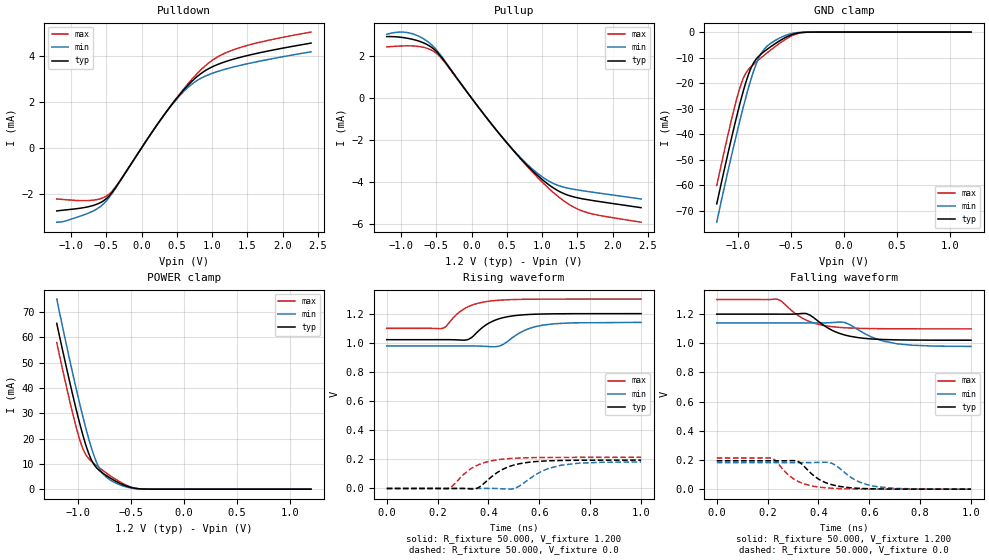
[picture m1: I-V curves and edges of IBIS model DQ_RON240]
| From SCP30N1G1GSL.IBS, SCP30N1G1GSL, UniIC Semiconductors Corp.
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|   Model DQ_RON240
[Model] DQ_RON240
Model_type I/O
Vinl =  0.500V
Vinh =  0.700V
Vmeas =  0.600V
Rref =  50.000
Vref =  0.600V
C_comp   1.373pF   1.353pF   1.403pF
[Model Spec]
Vinh   0.700V   0.670V   0.750V
Vinl   0.500V   0.470V   0.550V
Vmeas   0.600V   0.570V   0.650V
Vref   0.600V   0.570V   0.650V
Rref   50.000   NA   NA
[Temperature Range]   25.000   85.000   -40.000
[Voltage Range]   1.200V   1.140V   1.300V
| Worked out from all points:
|   slope of the pulldown table from 0 to 0.18 V, typ, clamps not added: 216 ohm
|   slope of the pullup table from 0 to 0.18 V, typ, clamps not added: 226 ohm
|   GND clamp passes 1 mA (typ) near -0.49 V on its own axis
|   POWER clamp passes 1 mA (typ) near -0.53 V on its own axis
|   rising waveform, R_fixture 50.000, V_fixture 1.200: 20-80 % time 94.3ps typ, 102ps min, 91.5ps max; typ from 1.02 V to 1.2 V
|   rising waveform, R_fixture 50.000, V_fixture 0.0: 20-80 % time 105ps typ, 116ps min, 100ps max; typ from 0 V to 0.194 V
|   falling waveform, R_fixture 50.000, V_fixture 1.200: 20-80 % time 114ps typ, 125ps min, 109ps max; typ from 1.2 V to 1.02 V
|   falling waveform, R_fixture 50.000, V_fixture 0.0: 20-80 % time 93.1ps typ, 101ps min, 90ps max; typ from 0.195 V to 0 V
[Pulldown]
|Voltage   I(typ)   I(min)   I(max)
-1.2V     -2.75mA    -3.242mA   -2.227mA
-719mV    -2.542mA   -2.803mA   -2.29mA
-571mV    -2.369mA   -2.53mA    -2.206mA
-460mV    -2.102mA   -2.169mA   -2.019mA
-349mV    -1.65mA    -1.672mA   -1.619mA
317mV     1.436mA    1.429mA    1.434mA
576mV     2.461mA    2.402mA    2.498mA
761mV     3.052mA    2.898mA    3.165mA
1.02V     3.574mA    3.286mA    3.872mA
1.279V    3.862mA    3.523mA    4.268mA
1.723V    4.195mA    3.827mA    4.656mA
2.4V      4.585mA    4.206mA    5.066mA
[Pullup]
|Voltage   I(typ)   I(min)   I(max)
-1.2V     2.921mA    3.034mA    2.433mA
-1.004V   2.89mA     3.136mA    2.474mA
-819mV    2.779mA    3.036mA    2.474mA
-634mV    2.552mA    2.717mA    2.37mA
-486mV    2.179mA    2.247mA    2.097mA
69mV      -308.7uA   -310.8uA   -304.4uA
439mV     -1.886mA   -1.882mA   -1.881mA
772mV     -3.149mA   -3.098mA   -3.19mA
1.031V    -3.961mA   -3.821mA   -4.099mA
1.29V     -4.522mA   -4.226mA   -4.851mA
1.549V    -4.78mA    -4.398mA   -5.349mA
2.4V      -5.216mA   -4.804mA   -5.907mA
[GND_clamp]
|Voltage   I(typ)   I(min)   I(max)
-1.2V     -67.26mA   -74.42mA   -60.1mA
-1.05V    -39.62mA   -46.47mA   -32.4mA
-1V       -31.05mA   -37.77mA   -24.37mA
-950mV    -23.16mA   -29.46mA   -18.1mA
-925mV    -19.62mA   -25.5mA    -16.02mA
-875mV    -13.89mA   -18.21mA   -13.48mA
-825mV    -10.4mA    -12.16mA   -11.61mA
-775mV    -8.365mA   -7.964mA   -9.852mA
-700mV    -6.001mA   -4.671mA   -7.319mA
-525mV    -1.587mA   -933.3uA   -2.208mA
-375mV    -90.13uA   -49.22uA   -132.9uA
1.2V      0A         0A         0A
[POWER_clamp]
|Voltage   I(typ)   I(min)   I(max)
-1.2V     65.51mA    75.11mA    57.91mA
-1.05V    37.38mA    45.87mA    29.99mA
-1V       28.74mA    36.73mA    21.95mA
-950mV    20.85mA    28.08mA    15.65mA
-925mV    17.34mA    24.01mA    13.56mA
-875mV    11.74mA    16.61mA    11.06mA
-825mV    8.457mA    10.65mA    9.317mA
-775mV    6.603mA    6.7mA      7.708mA
-725mV    5.177mA    4.492mA    6.178mA
-550mV    1.336mA    943.1uA    1.707mA
-400mV    85.95uA    67.55uA    91.19uA
1.2V      0A         0A         0A
[Ramp]
| variable   typ   min   max
dV/dt_r   0.117/0.106n   0.109/0.113n   0.128/0.101n
dV/dt_f   0.107/0.114n   96.921m/0.123n   0.121/0.109n
R_load = 50.000
[Rising Waveform]
R_fixture= 50.000
V_fixture= 1.200
V_fixture_min= 1.140
V_fixture_max= 1.300
|time   V(typ)   V(min)   V(max)
0s        1.021V     978.1mV    1.099V
222ps     1.021V     978.1mV    1.1V
282ps     1.019V     978.2mV    1.206V
321ps     1.023V     978.3mV    1.248V
418ps     1.149V     972.7mV    1.289V
451ps     1.169V     982.6mV    1.293V
542ps     1.192V     1.085V     1.298V
612ps     1.197V     1.121V     1.299V
728ps     1.2V       1.137V     1.3V
1ns       1.2V       1.14V      1.3V
[Rising Waveform]
R_fixture= 50.000
V_fixture= 0.0
V_fixture_min= 0.0
V_fixture_max= 0.0
|time   V(typ)   V(min)   V(max)
0s        74.14nV    239.6nV    42.63nV
237ps     13.37uV    -2.819uV   -1.917mV
258ps     104.2uV    -8.303uV   17.17mV
321ps     -1.88mV    676.2nV    123mV
355ps     1.071mV    93.81uV    158.4mV
452ps     127.8mV    -2.105mV   200.5mV
508ps     164.2mV    4.415mV    207.9mV
609ps     187.4mV    117.7mV    212.4mV
687ps     192.2mV    160mV      213.3mV
1ns       194.5mV    181.9mV    213.7mV
[Falling Waveform]
R_fixture= 50.000
V_fixture= 1.200
V_fixture_min= 1.140
V_fixture_max= 1.300
|time   V(typ)   V(min)   V(max)
0s        1.2V       1.14V      1.3V
240ps     1.2V       1.14V      1.301V
317ps     1.202V     1.14V      1.194V
352ps     1.204V     1.14V      1.159V
392ps     1.161V     1.14V      1.134V
452ps     1.091V     1.142V     1.114V
509ps     1.054V     1.139V     1.106V
617ps     1.029V     1.037V     1.101V
709ps     1.024V     996.8mV    1.1V
1ns       1.021V     978.5mV    1.099V
[Falling Waveform]
R_fixture= 50.000
V_fixture= 0.0
V_fixture_min= 0.0
V_fixture_max= 0.0
|time   V(typ)   V(min)   V(max)
0s        194.5mV    182.2mV    213.7mV
216ps     194.4mV    182.2mV    212.4mV
280ps     195.1mV    182.1mV    99.63mV
317ps     191.8mV    182mV      55.61mV
408ps     61.38mV    183.9mV    13.16mV
454ps     29.93mV    176.7mV    6.313mV
539ps     7.839mV    68.42mV    1.639mV
614ps     2.418mV    21.69mV    495.9uV
705ps     575uV      5.236mV    116.8uV
1ns       5.507uV    51.57uV    1.11uV
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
